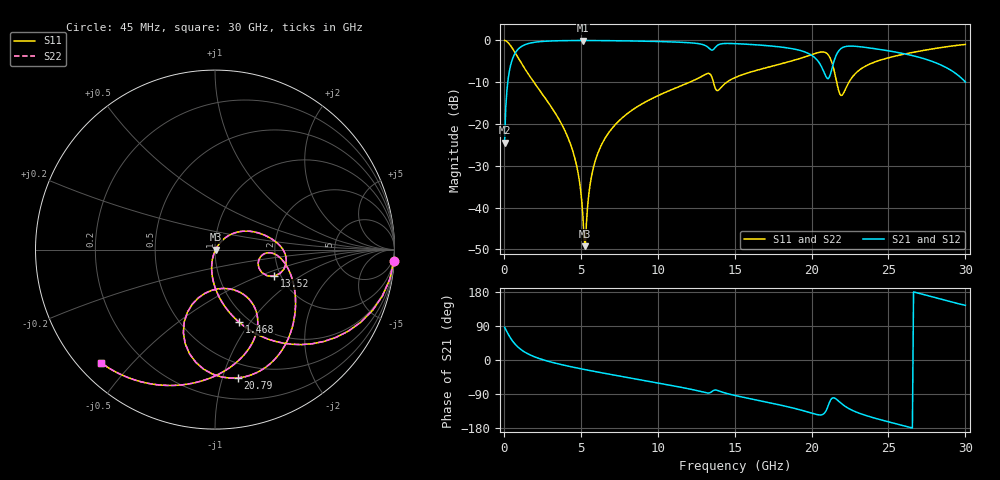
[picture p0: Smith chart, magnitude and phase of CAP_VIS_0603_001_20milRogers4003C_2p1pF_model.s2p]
! S-parameter model data by Modelithics Inc.  support@modelithics.com  813-866-6335  Tampa FL USA
! S-Parameter data specifications:
! Substrate: 20-mil Rogers 4003C, substrate thickness, H=0.508mm, Dielectric constant, Er=3.75
! PCB Mounting Pad Footprint: Pad width, PadW=0.90mm , Pad length, PadL=1.00mm , Pad gap, PadG (edge-to-edge)=1.00mm , Reference planes=3.0mm apart
! Created Wed Nov 18 13:20:21 2015
# hz S ma R 50
! 2 Port Network Data from SP1.SP block
! freq  magS11  angS11  magS21  angS21  magS12  angS12  magS22  angS22
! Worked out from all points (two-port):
!   401 points, 45 MHz to 30 GHz, reference 50 ohm
!   highest |S21| = -0.03 dB at 5.137 GHz (marker M1); lowest = -24.5 dB at 45 MHz (marker M2)
!   |S21| within 3 dB of the highest: 734.6 MHz to 19.74 GHz (19.01 GHz wide, 186 % of centre); 21.67 GHz to 25.8 GHz (4.124 GHz wide, 17.4 % of centre)
!   lowest |S11| = -49.2 dB at 5.287 GHz (marker M3), VSWR 1.01, Z = 50.3 - j0.0127 ohm
!   |S11| at or under -10 dB: 1.948 GHz to 12.08 GHz (10.13 GHz wide, 144 % of centre); 13.62 GHz to 14.49 GHz (866.6 MHz wide, 6.17 % of centre); 21.63 GHz to 22.43 GHz (797.1 MHz wide, 3.62 % of centre)
!   |S22| runs from -49.2 to 0.0 dB; largest |S21 - S12| = 0
!   S11 on the Smith chart (normalised r, x): 45 MHz: 1, -31; 1.468 GHz: 0.90, -0.89; 13.52 GHz: 1.85, -0.63; 20.79 GHz: 0.37, -1.12; 30 GHz: 0.07, -0.41
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4.5e7  0.9982 -3.7  0.0599 86.3  0.0599 86.3  0.9982 -3.7
4.94325e8  0.8325 -36.0  0.5534 54.0  0.5534 54.0  0.8325 -36.0
1.467862e9  0.4267 -71.6  0.9028 18.2  0.9028 18.2  0.4267 -71.6
4.163812e9  0.06868 -103.7  0.9945 -16.1  0.9945 -16.1  0.06868 -103.7
4.762912e9  0.02942 -105.4  0.9962 -21.2  0.9962 -21.2  0.02942 -105.4
5.062462e9  0.01182 -98.5  0.9964 -23.7  0.9964 -23.7  0.01182 -98.5
5.13735e9  0.007748 -90.6  0.9964 -24.3  0.9964 -24.3  0.007748 -90.6
5.287125e9  0.003448 -2.1  0.9964 -25.5  0.9964 -25.5  0.003448 -2.1
5.73645e9  0.02581 53.6  0.9959 -29.0  0.9959 -29.0  0.02581 53.6
6.485325e9  0.06312 52.0  0.9939 -34.7  0.9939 -34.7  0.06312 52.0
1.007992e10  0.221 27.4  0.9691 -61.2  0.9691 -61.2  0.221 27.4
1.352475e10  0.3613 -24.1  0.7641 -83.3  0.7641 -83.3  0.3613 -24.1
1.389919e10  0.2507 -12.8  0.876 -80.5  0.876 -80.5  0.2507 -12.8
1.50225e10  0.3589 -6.4  0.9148 -93.6  0.9148 -93.6  0.3589 -6.4
2.003996e10  0.6778 -57.3  0.6573 -140.6  0.6573 -140.6  0.6778 -57.3
2.078884e10  0.7263 -80.0  0.4246 -142.1  0.4246 -142.1  0.7263 -80.0
2.138794e10  0.4949 -110.9  0.5076 -99.8  0.5076 -99.8  0.4949 -110.9
2.198704e10  0.2212 -77.8  0.8154 -116.4  0.8154 -116.4  0.2212 -77.8
2.303546e10  0.4312 -57.1  0.8439 -139.5  0.8439 -139.5  0.4312 -57.1
2.505742e10  0.6233 -76.8  0.7471 -163.8  0.7471 -163.8  0.6233 -76.8
2.782826e10  0.7894 -106.6  0.5616 167.0  0.5616 167.0  0.7894 -106.6
3e10  0.8943 -135.0  0.3178 144.4  0.3178 144.4  0.8943 -135.0
